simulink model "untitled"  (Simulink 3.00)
settings: Solver=ode45  StartTime=0.0  StopTime=10.0  RelTol=1e-3
libraries: MIMO_lib x1

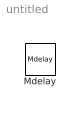
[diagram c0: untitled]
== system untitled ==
  Mdelay : MIMO_lib/Mdelay  Mdelay=abcd
